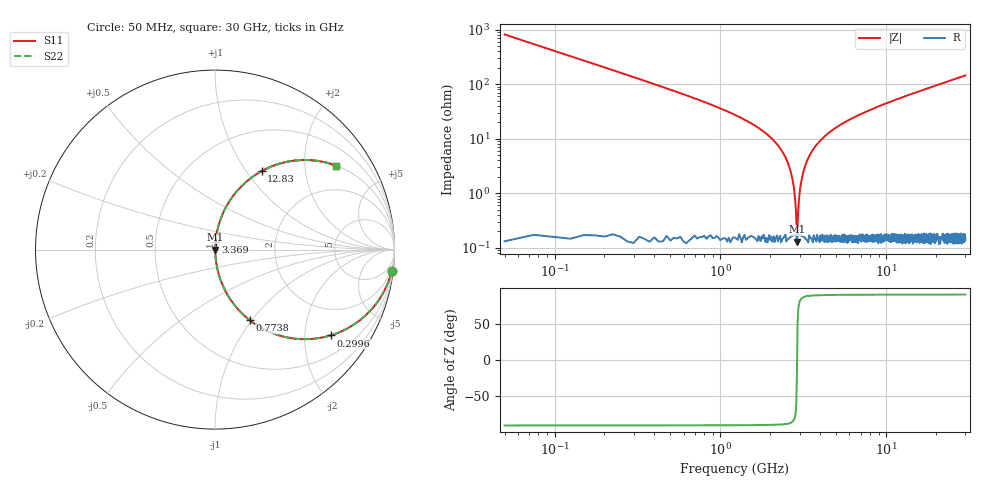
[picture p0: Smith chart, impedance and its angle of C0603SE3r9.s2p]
!	AVX Thin Film Operation 	Date: April 2014
!	Description: Accu-P® Series, Thin Film  SMD RF Capacitor
!	Part Number: 06031J3R9ABSTR
# MHZ S MA R 50
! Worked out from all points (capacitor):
!   1201 points, 50 MHz to 30 GHz, reference 50 ohm
!   read as one part in series: C = 3.9 pF near 199.8 MHz
!   lowest |Z| = 129 mohm at 2.895 GHz (marker M1)
!   series resonance near 2.899 GHz, so ESL is about 770 pH
!   S11 on the Smith chart (normalised r, x): 50 MHz: 1, -16; 299.6 MHz: 1.00, -2.70; 773.8 MHz: 1.00, -0.98; 3.369 GHz: 1.00, +0.08; 12.83 GHz: 1.00, +1.18; 30 GHz: 1.00, +2.89
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50  0.993 -7.0  0.122 83.0  0.122 83.0  0.993 -7.0
299.583  0.803 -36.6  0.596 53.4  0.596 53.4  0.803 -36.6
524.208  0.601 -52.9  0.798 36.9  0.798 36.9  0.601 -52.9
773.792  0.439 -63.8  0.897 26.1  0.897 26.1  0.439 -63.8
1322.875  0.237 -75.9  0.97 13.7  0.97 13.7  0.237 -75.9
2321.208  0.063 -85.0  0.997 3.6  0.997 3.6  0.063 -85.0
2595.75  0.031 -85.5  0.998 1.8  0.998 1.8  0.031 -85.5
2695.583  0.02 -84.6  0.998 1.2  0.998 1.2  0.02 -84.6
2795.417  0.01 -81.1  0.998 0.6  0.998 0.6  0.01 -81.1
2895.25  0.001534 -12.5  0.999 0.0  0.999 0.0  0.001534 -12.5
2995.083  0.009322 80.2  0.998 -0.5  0.998 -0.5  0.009322 80.2
3144.833  0.023 85.0  0.998 -1.3  0.998 -1.3  0.023 85.0
3369.458  0.042 85.5  0.998 -2.4  0.998 -2.4  0.042 85.5
3993.417  0.091 83.8  0.994 -5.2  0.994 -5.2  0.091 83.8
5041.667  0.162 80.2  0.985 -9.3  0.985 -9.3  0.162 80.2
6988.417  0.27 74.0  0.961 -15.7  0.961 -15.7  0.27 74.0
10058.29  0.408 65.7  0.911 -24.1  0.911 -24.1  0.408 65.7
12828.67  0.508 59.3  0.86 -30.6  0.86 -30.6  0.508 59.3
15025  0.574 54.8  0.817 -35.1  0.817 -35.1  0.574 54.8
20016.67  0.689 46.4  0.724 -43.5  0.724 -43.5  0.689 46.4
25033.29  0.768 39.8  0.64 -50.1  0.64 -50.1  0.768 39.8
30000  0.822 34.7  0.569 -55.2  0.569 -55.2  0.822 34.7
